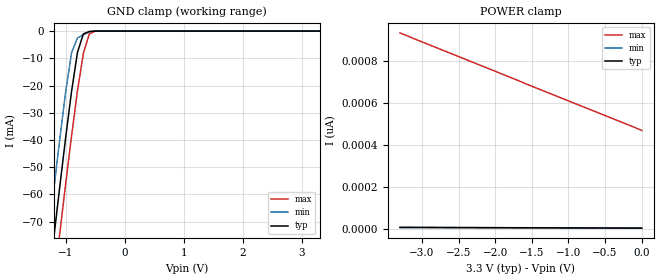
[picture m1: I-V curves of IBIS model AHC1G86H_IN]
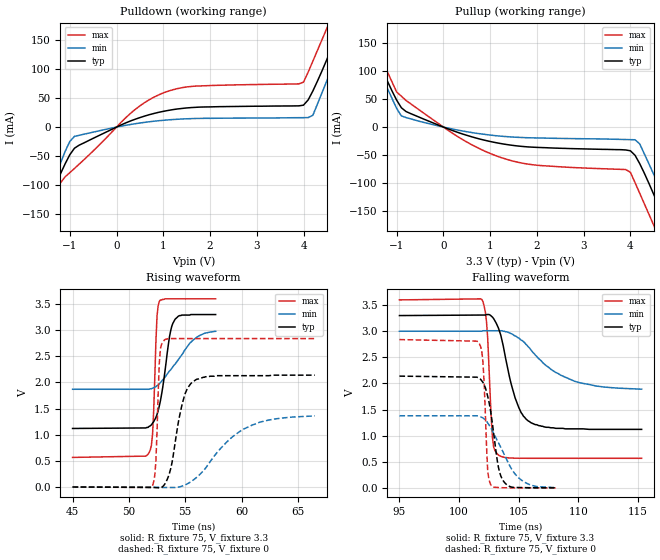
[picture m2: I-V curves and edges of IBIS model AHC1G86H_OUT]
| TEXAS INSTRUMENTS INCORPORATED
| Standard Linear and Logic Group
| IBIS Model of SN74AHC1G86H
| SINGLE 2-INPUT EXCLUSIVE-OR GATE
| CMPAK-5 5-pin (DCK) Package
[IBIS Ver]   2.1
[Comment Char]  |_char
[File name]   ul86_3c.ibs
[File Rev]   2.0
[Date]   May 11, 2000
[Source]   Data created from SPICE simulations at Hitachi,Ltd.
[Notes]   The following is an IBIS List for the AHC1G86H.
|   Please contact sllibis@ti.com with questions and
|   comments concerning SLL IBIS models.
[Disclaimer] Property of Texas Instruments Incorporated.  Unauthorized
   reproduction and/or distribution is strictly prohibited.
   This product is protected under copyright law.
   Created 2000, (C) Copyright 2000, Texas Instruments Inc.,
   All Rights Reserved.
   UNLESS THERE IS A SIGNED, WRITTEN AGREEMENT TO THE
   CONTRARY, TEXAS INSTRUMENTS () IS PROVIDING THE IBIS
   MODELS  AND WITHOUT ANY WARRANTY, EXPRESSED OR
   IMPLIED.  TI assumes no liability for:
   1) the accuracy of the IBIS models provided to your
   company;
   2) the proper functioning of these IBIS Models in your
   design or for any resulting applications; or
   3) infringement of patents, copyrights or intellectual
   property rights resulting from your use of these IBIS
   models.
   TI provides IBIS Models as a service to our customers.
   You and your company shall not distribute, sell or give
   these models to anyone else without prior written
   permission from TI.
   TI reserves the right to make changes to our products or
   to discontinue any semiconductor product or service
   without notice, and advises our customers to obtain the
   latest version of relevant information to verify, before
   placing orders, that the information being relied on is
   current.
   Please be aware that your receipt and use of the IBIS
   information provided shall serve as acceptance of these
   terms and conditions.  If you do not accept these terms,
   you should return or destroy the IBIS models and any
   other accompanying information immediately.
|   Component AHC1G86H
[Component]   AHC1G86H
[Manufacturer]   Hitachi, Ltd.
[Package]
|   typ   min   max
R_pkg   0.090   0.051   0.105
L_pkg   1.500nH   0.940nH   1.700nH
C_pkg   0.170pF   0.110pF   0.360pF
[Pin]   signal_name   model_name   R_pin   L_pin   C_pin
1   A   AHC1G86H_IN   0.098   1.590nH   0.110pF
2   B   AHC1G86H_IN   0.051   0.940nH   0.170pF
3   GND   GND   0.092   1.590nH   0.360pF
4   Y   AHC1G86H_OUT   0.105   1.700nH   0.110pF
5   VCC   POWER   0.104   1.690nH   0.110pF
| Models and submodels in the file (2): AHC1G86H_IN (Input), AHC1G86H_OUT (Output)
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|   Model AHC1G86H_IN
[Model]   AHC1G86H_IN
Model_type  Input
Polarity   Inverting
Vinl = 0.99
Vinh = 2.31
| variable   typ   min   max
C_comp   1.80pF   1.73pF   1.97pF
[Temperature Range]   25   85   -40
[Voltage Range]   3.3   3.0   3.6
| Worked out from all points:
|   GND clamp passes 1 mA (typ) near -0.70 V on its own axis
[GND Clamp]
|   Voltage   I(typ)   I(min)   I(max)
-3.3V     -486mA     -469mA     -503mA
-1.3V     -94.6mA    -76.9mA    -112mA
-1.2V     -75.8mA    -58.1mA    -93.1mA
-1.1V     -57.3mA    -39.8mA    -74.5mA
-1V       -39.2mA    -22.4mA    -56.2mA
-900mV    -22.2mA    -7.98mA    -38.6mA
-800mV    -7.87mA    -2.53mA    -22mA
-700mV    -1.03mA    -1.34mA    -8.2mA
-600mV    -206uA     -154uA     -1.06mA
-500mV    -11.2uA    -2.6uA     -57.2uA
3.3V      3.55pA     3.3pA      469pA
[POWER Clamp]
|   Voltage   I(typ)   I(min)   I(max)
-3.3V     7pA        6.6pA      934pA
-1.6V     5.23pA     4.9pA      694pA
-100mV    3.66pA     3.4pA      484pA
0V        3.55pA     3.3pA      469pA
|   Model AHC1G86H_OUT
[Model]   AHC1G86H_OUT
Model_type  Output
Polarity   Inverting
Vmeas = 1.65
Cref = 15pf
| variable   typ   min   max
C_comp   3.84pF   3.72pF   3.96pF
[Temperature Range]   25   85   -40
[Voltage Range]   3.3   3.0   3.6
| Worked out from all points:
|   slope of the pulldown table from 0 to 0.495 V, typ, clamps not added: 30.4 ohm
|   slope of the pullup table from 0 to 0.495 V, typ, clamps not added: 34 ohm
|   rising waveform, R_fixture 75, V_fixture 3.3: 20-80 % time 890ps typ, 2.27ns min, 304ps max; typ from 1.12 V to 3.3 V
|   falling waveform, R_fixture 75, V_fixture 3.3: 20-80 % time 1.42ns typ, 3.47ns min, 380ps max; typ from 3.3 V to 1.12 V
|   falling waveform, R_fixture 75, V_fixture 0: 20-80 % time 834ps typ, 1.88ns min, 313ps max; typ from 2.14 V to 0 V
|   rising waveform, R_fixture 75, V_fixture 0: 20-80 % time 1.1ns typ, 3.58ns min, 271ps max; typ from 0 V to 2.14 V
[Pulldown]
|   Voltage   I(typ)   I(min)   I(max)
-3.3V     -489mA     -473mA     -506mA
-1.8V     -194mA     -179mA     -211mA
-1.6V     -156mA     -142mA     -173mA
-1.2V     -81mA      -62.6mA    -96.6mA
-900mV    -36.6mA    -16.1mA    -71.6mA
1V        27.2mA     11.7mA     59.1mA
3.9V      36.7mA     16.2mA     74.7mA
4.1V      47mA       16.4mA     95.1mA
4.5V      117mA      80.2mA     171mA
4.8V      174mA      137mA      229mA
5V        213mA      175mA      268mA
6.6V      528mA      491mA      584mA
[Pullup]
|   Voltage   I(typ)   I(min)   I(max)
-3.3V     491mA      474mA      508mA
-1.8V     196mA      179mA      214mA
-1.6V     157mA      141mA      175mA
-1V       47.9mA     33.1mA     62.4mA
-900mV    34.5mA     20mA       55.1mA
1.2V      -29mA      -16mA      -53.4mA
3.9V      -40.8mA    -22.2mA    -75.7mA
4.2V      -65.2mA    -30mA      -118mA
4.5V      -120mA     -84.4mA    -175mA
4.8V      -177mA     -138mA     -233mA
5V        -216mA     -177mA     -272mA
6.6V      -533mA     -494mA     -589mA
[Ramp]
| variable   typ   min   max
dV/dt_r   1.28E+00/1.09E-09   8.26E-01/3.68E-09   1.71E+00/2.70E-10
dV/dt_f   1.31E+00/1.41E-09   6.74E-01/3.54E-09   1.82E+00/3.80E-10
R_load = 75
[Rising Waveform]
R_fixture = 75
V_fixture = 3.3
V_fixture_min = 3.0
V_fixture_max = 3.6
|   Time   V(typ)   V(min)   V(max)
45ns      1.12V      1.87V      566mV
51.7ns    1.14V      1.87V      627mV
52.1ns    1.22V      1.89V      1.01V
52.2ns    1.25V      1.9V       1.45V
52.5ns    1.39V      1.94V      3.28V
52.7ns    1.55V      1.97V      3.55V
53.6ns    2.87V      2.22V      3.6V
54.1ns    3.21V      2.35V      3.6V
55.8ns    3.3V       2.83V      3.6V
57.7ns    3.3V       2.98V      3.6V
[Falling Waveform]
R_fixture = 75
V_fixture = 3.3
V_fixture_min = 3.0
V_fixture_max = 3.6
|   Time   V(typ)   V(min)   V(max)
95ns      3.3V       3V         3.6V
101.9ns   3.31V      3V         3.61V
102.3ns   3.32V      3.01V      3.18V
102.8ns   3.27V      3.01V      957mV
103ns     3.2V       3.01V      716mV
103.4ns   2.99V      3.01V      615mV
104.7ns   1.72V      2.91V      569mV
105.8ns   1.28V      2.7V       566mV
109.7ns   1.13V      2.04V      566mV
115.3ns   1.12V      1.89V      566mV
[Falling Waveform]
R_fixture = 75
V_fixture = 0
|   Time   V(typ)   V(min)   V(max)
95ns      2.14V      1.38V      2.84V
101.6ns   2.11V      1.38V      2.79V
102ns     2.02V      1.34V      2.41V
102.1ns   1.97V      1.32V      2.01V
102.4ns   1.75V      1.24V      317mV
102.7ns   1.38V      1.13V      42.3mV
103.3ns   391mV      863mV      5.82mV
103.8ns   104mV      632mV      1.93mV
105.4ns   4.55mV     121mV      85uV
108.1ns   439uV      4.7mV      -9uV
[Rising Waveform]
R_fixture = 75
V_fixture = 0
|   Time   V(typ)   V(min)   V(max)
45ns      0V         0V         0V
52ns      -7.71mV    -2.5mV     -9.67mV
52.4ns    -11.9mV    -5.32mV    501mV
52.7ns    -16.3mV    -7.69mV    2.37V
52.8ns    -15.5mV    -8.32mV    2.65V
53.2ns    60.4mV     -9.57mV    2.82V
54.7ns    1.56V      15mV       2.84V
55.6ns    2V         115mV      2.84V
60.1ns    2.13V      1.1V       2.84V
66.5ns    2.14V      1.36V      2.84V
